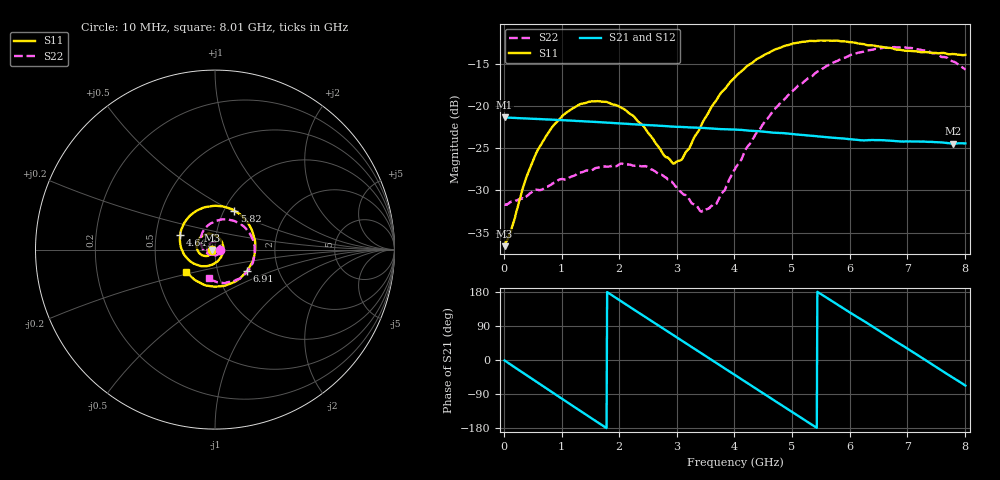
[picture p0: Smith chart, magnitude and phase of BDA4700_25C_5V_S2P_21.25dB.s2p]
!Agilent Technologies,E5071B,MY42404982,A.09.10
!Date: Mon Oct 20 13:37:03 2025
!Data & Calibration Information:
!Freq	S11:SOLT2(ON)	S21:SOLT2(ON)	S12:SOLT2(ON)	S22:SOLT2(ON)
# Hz S RI R 50
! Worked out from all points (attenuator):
!   801 points, 10 MHz to 8.01 GHz, reference 50 ohm
!   highest |S21| = -21.34 dB at 10 MHz (marker M1); lowest = -24.5 dB at 7.8 GHz (marker M2)
!   lowest |S11| = -36.6 dB at 10 MHz (marker M3), VSWR 1.03, Z = 48.5 - j0.134 ohm
!   |S11| at or under -10 dB: start of sweep to end of sweep
!   |S22| runs from -32.5 to -13.0 dB; largest |S21 - S12| = 0.00069
!   S11 on the Smith chart (normalised r, x): 10 MHz: 0.97, -0.00; 4.64 GHz: 0.67, +0.11; 5.82 GHz: 1.12, +0.52; 6.91 GHz: 1.38, -0.35; 8.01 GHz: 0.71, -0.18
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1e7  -0.0147 -0.00138  0.0857 -0.00184  0.0857 -0.00195  0.026 -0.000842
1.4e8  -0.0163 -0.0103  0.0823 -0.0215  0.0823 -0.0215  0.0264 -0.00672
3.8e8  -0.0262 -0.0264  0.0655 -0.0532  0.0655 -0.0532  0.0213 -0.0196
5.9e8  -0.0425 -0.0354  0.0414 -0.0728  0.0414 -0.0728  0.0134 -0.029
1e9  -0.083 -0.0237  -0.0167 -0.0808  -0.0167 -0.0809  -0.0149 -0.0339
1.35e9  -0.1024 0.0133  -0.0593 -0.0556  -0.0593 -0.0557  -0.0365 -0.0176
2.07e9  -0.0425 0.0865  -0.0691 0.0377  -0.0691 0.0378  -0.0301 0.0339
2.68e9  0.0382 0.0429  -0.00152 0.0764  -0.00151 0.0765  0.0139 0.0372
2.92e9  0.046 0.00287  0.0289 0.0698  0.0289 0.0698  0.0254 0.0247
3.05e9  0.0428 -0.0206  0.0434 0.0615  0.0431 0.0616  0.0278 0.0146
3.44e9  -0.00599 -0.0788  0.0711 0.0212  0.0712 0.0212  0.0184 -0.0151
3.69e9  -0.0579 -0.0921  0.0726 -0.0101  0.0726 -0.0103  -0.000145 -0.0264
4.01e9  -0.1298 -0.0704  0.056 -0.046  0.056 -0.046  -0.0331 -0.0261
4.64e9  -0.1936 0.082  -0.0141 -0.0683  -0.0141 -0.0683  -0.0797 0.0423
5.35e9  -0.0492 0.2376  -0.0658 -0.0101  -0.0659 -0.0103  -0.0152 0.1494
5.82e9  0.1081 0.217  -0.0517 0.0385  -0.0516 0.0386  0.0904 0.1642
6.24e9  0.2062 0.1077  -0.0147 0.0609  -0.014 0.061  0.1799 0.1074
6.68e9  0.2154 -0.0482  0.0303 0.0545  0.0304 0.0545  0.2209 -0.00213
6.91e9  0.1768 -0.1204  0.0479 0.0387  0.0481 0.0386  0.2132 -0.0665
7.35e9  0.0445 -0.2034  0.0612 -0.00373  0.0613 -0.0039  0.1388 -0.1612
7.8e9  -0.1084 -0.1715  0.0408 -0.0439  0.0408 -0.044  0.0176 -0.1821
8.01e9  -0.1591 -0.1222  0.023 -0.0555  0.0231 -0.0555  -0.0327 -0.1607
